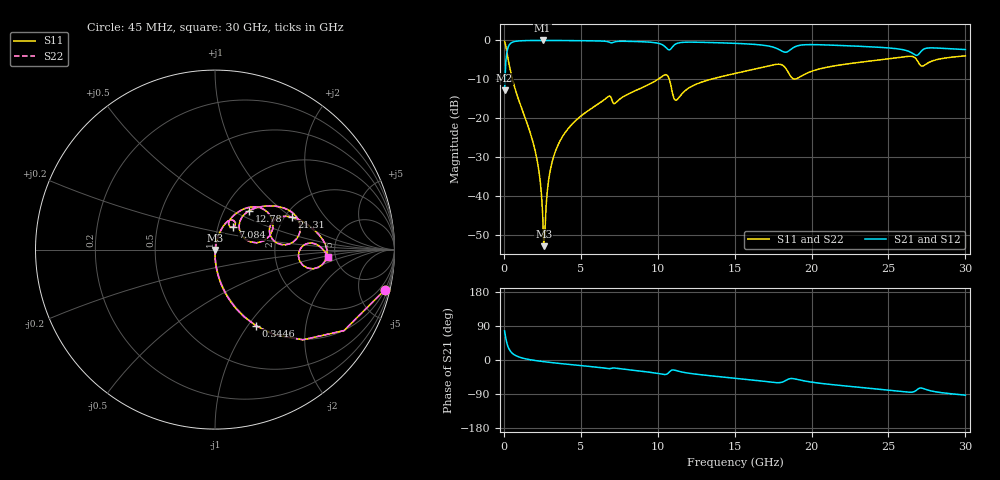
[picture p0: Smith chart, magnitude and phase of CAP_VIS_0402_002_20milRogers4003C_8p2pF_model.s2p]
! S-parameter model data by Modelithics Inc.  support@modelithics.com  813-866-6335  Tampa FL USA
! S-Parameter data specifications:
! Substrate: 20-mil Rogers 4003C, substrate thickness, H=0.508mm, Dielectric constant, Er=3.75
! PCB Mounting Pad Footprint: Pad width, PadW=0.50mm , Pad length, PadL=0.50mm , Pad gap, PadG (edge-to-edge)=0.40mm , Reference planes=1.4mm apart
! Created Wed Nov 18 12:50:01 2015
# hz S ma R 50
! 2 Port Network Data from SP1.SP block
! freq  magS11  angS11  magS21  angS21  magS12  angS12  magS22  angS22
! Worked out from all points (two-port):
!   401 points, 45 MHz to 30 GHz, reference 50 ohm
!   highest |S21| = -0.02 dB at 2.516 GHz (marker M1); lowest = -12.9 dB at 45 MHz (marker M2)
!   |S21| within 3 dB of the highest: 192.9 MHz to 18.24 GHz (18.05 GHz wide, 196 % of centre); 18.36 GHz to 26.42 GHz (8.065 GHz wide, 36 % of centre)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
!   lowest |S11| = -53.0 dB at 2.591 GHz (marker M3), VSWR 1.00, Z = 50.2 - j0.149 ohm
!   |S11| at or under -10 dB: 553.4 MHz to 10.02 GHz (9.469 GHz wide, 179 % of centre); 10.75 GHz to 13.47 GHz (2.717 GHz wide, 22.4 % of centre)
!   |S22| runs from -53.0 to -0.2 dB; largest |S21 - S12| = 0
!   S11 on the Smith chart (normalised r, x): 45 MHz: 0.99, -8.53; 344.6 MHz: 0.99, -1.09; 7.084 GHz: 1.18, +0.30; 12.78 GHz: 1.30, +0.61; 21.31 GHz: 2.17, +1.00; 30 GHz: 4.35, -0.61
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4.5e7  0.9739 -13.2  0.2271 76.8  0.2271 76.8  0.9739 -13.2
3.4455e8  0.482 -61.7  0.8755 28.2  0.8755 28.2  0.482 -61.7
7.93875e8  0.2155 -78.7  0.9755 11.1  0.9755 11.1  0.2155 -78.7
1.992075e9  0.04079 -88.9  0.9975 -1.1  0.9975 -1.1  0.04079 -88.9
2.291625e9  0.0197 -87.9  0.998 -2.9  0.998 -2.9  0.0197 -87.9
2.516288e9  0.005973 -76.8  0.9981 -4.0  0.9981 -4.0  0.005973 -76.8
2.591175e9  0.002245 -41.3  0.9981 -4.4  0.9981 -4.4  0.002245 -41.3
2.965612e9  0.01891 77.9  0.9978 -6.2  0.9978 -6.2  0.01891 77.9
3.34005e9  0.03701 78.9  0.9972 -7.9  0.9972 -7.9  0.03701 78.9
5.062462e9  0.1083 73.5  0.9912 -15.0  0.9912 -15.0  0.1083 73.5
7.084425e9  0.1581 51.6  0.9409 -21.0  0.9409 -21.0  0.1581 51.6
1.007992e10  0.3218 47.8  0.9129 -36.1  0.9129 -36.1  0.3218 47.8
1.060414e10  0.3577 25.7  0.7832 -36.9  0.7832 -36.9  0.3577 25.7
1.120324e10  0.1698 32.8  0.9055 -27.9  0.9055 -27.9  0.1698 32.8
1.277588e10  0.2865 48.7  0.9455 -38.8  0.9455 -38.8  0.2865 48.7
1.50225e10  0.3747 40.4  0.9166 -48.1  0.9166 -48.1  0.3747 40.4
1.846732e10  0.3931 3.9  0.7199 -50.9  0.7199 -50.9  0.3931 3.9
2.003996e10  0.4026 26.7  0.8824 -58.7  0.8824 -58.7  0.4026 26.7
2.131305e10  0.4634 23.0  0.8686 -64.9  0.8686 -64.9  0.4634 23.0
2.505742e10  0.5797 8.9  0.7983 -79.6  0.7983 -79.6  0.5797 8.9
2.685472e10  0.5569 -11.1  0.6426 -78.5  0.6426 -78.5  0.5569 -11.1
3e10  0.6323 -3.8  0.7621 -92.8  0.7621 -92.8  0.6323 -3.8
